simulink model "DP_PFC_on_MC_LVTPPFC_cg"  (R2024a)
settings: Solver=FixedStepDiscrete  StartTime=0.0  StopTime=0.2  FixedStep=10e-6  RelTol=1e-3  EnableMultiTasking=on
model workspace (MAT data in the model file):
  Freq = 100
  Phas = 0
  SinFreq_1 = 250
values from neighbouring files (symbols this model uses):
  ADC = ADCType.Noise    [TotemPole_PFCData.m]
  Control = ControlType.Simple    [TotemPole_PFCData.m]
  Tsc_slow = 0.01    [TotemPole_PFCData.m]
undefined symbols (not defined in the file or in its folder): a, A0, A8, AD1, AD2, AD3, AD4, AD5, address, also, AN11, AN2, AN3, AN5, AN6, AppData, as, B0, B10, B11, B7, B8, below, bin2dec, bit, bits, BOR, C, C6, C7, C9, cause, characters, Code, Communicate, contains, counter, D, D4, Data, data, dead, default, Detailed, deviced, disasserted, DS70005539, dsPIC33AK128MC106, EC, ECIO, ensure, events, Family, faster, Floating, fulll, highest, HS, HS3, I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
libraries: MCHP_Blockset x16, simulink x4, dspswit3 x1
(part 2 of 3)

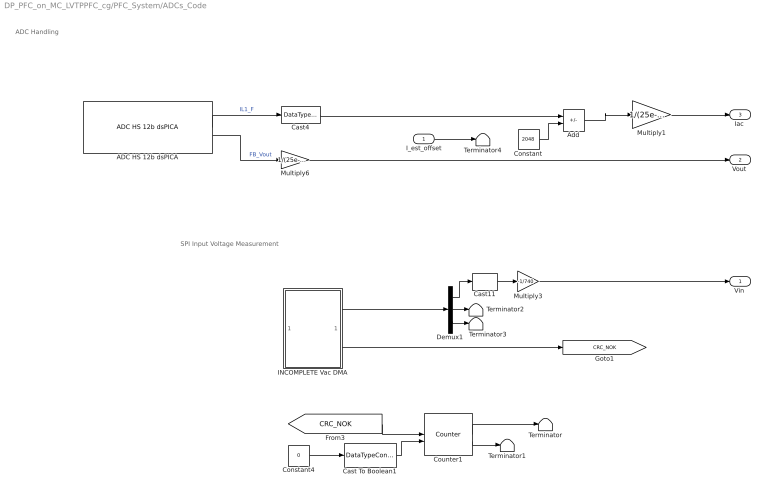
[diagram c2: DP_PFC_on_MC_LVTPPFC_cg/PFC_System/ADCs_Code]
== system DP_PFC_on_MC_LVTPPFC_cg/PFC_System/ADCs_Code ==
  note: ADC Handling
  note: SPI Input Voltage Measurement
  I_est_offset : Inport
  ADC HS 12b dsPICA : MCHP_Blockset/Analog IO/ADC HS 12b dsPICA  ADCREF=ADC 1 and ADC 2  ADC1_refChannel=0 (highest priority)  ADC2_refChannel=0 (highest priority)  ADC3_refChannel=0 (highest priority)  ADC4_refChannel=0 (highest priority)  ADC5_refChannel=Not used  CALRATE=once at startup  VREF_RNG=3.0V to 3.6V  BUFEN=on  info=0  SampleTime=10e-6  MCHP_PORT={ADC1_seq0.0}{ADC1B8}15:2:B8;{ADC2_seq0.0}{ADC2A0}15:2:A0;{ADC1_seq0.0}{ADC1B8}15:2:B8;{ADC2_seq0.0}{ADC2A0}15:2:A0;  MCHP_MASTERLINK=TotemPole_PFC_CodeGen/PFC_System/Control Variant /Microchip Master1  MCHP_CRC=34192788  ADC_Synchronisation=Triggered by custom source  ADC_Trig_TXT=PWM1_Trg1  ADC_TrigTimeStep=on  TrigSource_seq0=Dynamic Options  TrigSource_seq0_TXT=PWM1 adc trig 0  SampleTime_seq0_Tad=Dynamic Options  SampleTime_seq0_Tad_TXT="4.5 Tad  = 56.2ns  -  Rin < 5.2 kOhm"  ADC1_seq0=Dynamic Options  ADC1_seq0_TXT=AD1 AN11 / B8 / Pin[23]  ADC1_seq0_align=Right aligned  ADC1_seq0_overSampling=x1 (12 bits)  ADC2_seq0=Dynamic Options  ADC2_seq0_TXT=AD2 AN6 / A0 / Pin[1]  ADC2_seq0_align=Right aligned  ADC2_seq0_overSampling=x1 (12 bits)  ADC3_seq0=Dynamic Options  ADC3_seq0_TXT=AD3 AN5 / A0 / Pin[1]  ADC3_seq0_align=Left aligned  ADC3_seq0_overSampling=x1 (12 bits)  ADC4_seq0=Dynamic Options  ADC4_seq0_TXT=AD4 AN2 / B7 / Pin[30]  ADC4_seq0_align=Right aligned  ADC4_seq0_overSampling=x256 (16 bits)  ADC5_seq0=Dynamic Options  ADC5_seq0_TXT=AD5 AN3 / A8 / Pin[7]  ADC5_seq0_align=Right aligned  ADC5_seq0_overSampling=x256 (16 bits)  ADC1_seq0_1=Dynamic Options  ADC1_seq0_1_TXT=Not Used  ADC1_seq0_1_align=Right aligned  ADC1_seq0_1_overSampling=x1 (12 bits)  ADC2_seq0_1=Dynamic Options  ADC2_seq0_1_TXT=Not Used  ADC2_seq0_1_align=Right aligned  ADC2_seq0_1_overSampling=x1 (12 bits)  ADC3_seq0_1=Dynamic Options  ADC3_seq0_1_TXT=Not Used  ADC3_seq0_1_align=Right aligned  ADC3_seq0_1_overSampling=x1 (12 bits)  ADC4_seq0_1=Dynamic Options  ADC4_seq0_1_TXT=Not Used  ADC4_seq0_1_align=Right aligned  ADC4_seq0_1_overSampling=x1 (12 bits)  ADC5_seq0_1=Dynamic Options  ADC5_seq0_1_TXT=Not Used  ADC5_seq0_1_align=Right aligned  ADC5_seq0_1_overSampling=x1 (12 bits)  ADC1_seq0_2=Dynamic Options  ADC1_seq0_2_TXT=Not Used  ADC1_seq0_2_align=Right aligned  ADC1_seq0_2_overSampling=x1 (12 bits)  ADC2_seq0_2=Dynamic Options  ADC2_seq0_2_TXT=Not Used  ADC2_seq0_2_align=Right aligned  ADC2_seq0_2_overSampling=x1 (12 bits)  ADC3_seq0_2=Dynamic Options  ADC3_seq0_2_TXT=Not Used  ADC3_seq0_2_align=Right aligned  ADC3_seq0_2_overSampling=x1 (12 bits)  ADC4_seq0_2=Dynamic Options  ADC4_seq0_2_TXT=Not Used  ADC4_seq0_2_align=Right aligned  ADC4_seq0_2_overSampling=x1 (12 bits)  ADC5_seq0_2=Dynamic Options  ADC5_seq0_2_TXT=Not Used  ADC5_seq0_2_align=Right aligned  ADC5_seq0_2_overSampling=x1 (12 bits)  ADC1_seq0_3=Dynamic Options  ADC1_seq0_3_TXT=Not Used  ADC1_seq0_3_align=Right aligned  ADC1_seq0_3_overSampling=x1 (12 bits)  ADC2_seq0_3=Dynamic Options  ADC2_seq0_3_TXT=Not Used  ADC2_seq0_3_align=Right aligned  ADC2_seq0_3_overSampling=x1 (12 bits)  ADC3_seq0_3=Dynamic Options  ADC3_seq0_3_TXT=Not Used  ADC3_seq0_3_align=Right aligned  ADC3_seq0_3_overSampling=x1 (12 bits)  ADC4_seq0_3=Dynamic Options  ADC4_seq0_3_TXT=Not Used  ADC4_seq0_3_align=Right aligned  ADC4_seq0_3_overSampling=x1 (12 bits)  ADC5_seq0_3=Dynamic Options  ADC5_seq0_3_TXT=Not Used  ADC5_seq0_3_align=Right aligned  ADC5_seq0_3_overSampling=x1 (12 bits)  ADC1_seq0_4=Dynamic Options  ADC1_seq0_4_TXT=Not Used  ADC1_seq0_4_align=Right aligned  ADC1_seq0_4_overSampling=x1 (12 bits)  ADC2_seq0_4=Dynamic Options  ADC2_seq0_4_TXT=Not Used  ADC2_seq0_4_align=Right aligned  ADC2_seq0_4_overSampling=x1 (12 bits)  ADC3_seq0_4=Dynamic Options  ADC3_seq0_4_TXT=Not Used  ADC3_seq0_4_align=Right aligned  ADC3_seq0_4_overSampling=x1 (12 bits)  ADC4_seq0_4=Dynamic Options  ADC4_seq0_4_TXT=Not Used  ADC4_seq0_4_align=Right aligned  ADC4_seq0_4_overSampling=x1 (12 bits)  ADC5_seq0_4=Dynamic Options  ADC5_seq0_4_TXT=Not Used  ADC5_seq0_4_align=Right aligned  ADC5_seq0_4_overSampling=x1 (12 bits)  ADC1_seq0_5=Dynamic Options  ADC1_seq0_5_TXT=Not Used  ADC1_seq0_5_align=Right aligned  ADC1_seq0_5_overSampling=x1 (12 bits)  ADC2_seq0_5=Dynamic Options  ADC2_seq0_5_TXT=Not Used  ADC2_seq0_5_align=Right aligned  ADC2_seq0_5_overSampling=x1 (12 bits)  ADC3_seq0_5=Dynamic Options  ADC3_seq0_5_TXT=Not Used  ADC3_seq0_5_align=Right aligned  ADC3_seq0_5_overSampling=x1 (12 bits)  ADC4_seq0_5=Dynamic Options  ADC4_seq0_5_TXT=Not Used  ADC4_seq0_5_align=Right aligned  ADC4_seq0_5_overSampling=x1 (12 bits)  ADC5_seq0_5=Dynamic Options  ADC5_seq0_5_TXT=Not Used  ADC5_seq0_5_align=Right aligned  ADC5_seq0_5_overSampling=x1 (12 bits)  ADC_TRG2_ACCBRST_seq0=Burst - not interruptible  ADC1_NINSEL_seq0=Dynamic Options  ADC1_NINSEL_seq0_TXT=Vss - single ended (unsigned)  ADC2_NINSEL_seq0=Dynamic Options  ADC2_NINSEL_seq0_TXT=Vss - single ended (unsigned)  ADC3_NINSEL_seq0=Dynamic Options  ADC3_NINSEL_seq0_TXT=Vss - single ended (unsigned)  ADC4_NINSEL_seq0=Dynamic Options  ADC4_NINSEL_seq0_TXT=Vss - single ended (unsigned)  ADC5_NINSEL_seq0=Dynamic Options  ADC5_NINSEL_seq0_TXT=Vss - single ended (unsigned)  TrigTimeStep_seq0=on  info_seq0=0  TrigSource_seq1=Dynamic Options  TrigSource_seq1_TXT=after previous sequence  SampleTime_seq1_Tad=Dynamic Options  SampleTime_seq1_Tad_TXT="0.5 Tad  = 6.25ns  -  Rin < 0 kOhm"  ADC1_seq1=Dynamic Options  ADC1_seq1_TXT=Not Used  ADC1_seq1_align=Right aligned  ADC1_seq1_overSampling=x1 (12 bits)  ADC2_seq1=Dynamic Options  ADC2_seq1_TXT=Not Used  ADC2_seq1_align=Right aligned  ADC2_seq1_overSampling=x1 (12 bits)  ADC3_seq1=Dynamic Options  ADC3_seq1_TXT=Not Used  ADC3_seq1_align=Right aligned  ADC3_seq1_overSampling=x1 (12 bits)  ADC4_seq1=Dynamic Options  ADC4_seq1_TXT=Not Used  ADC4_seq1_align=Right aligned  ADC4_seq1_overSampling=x1 (12 bits)  ADC5_seq1=Dynamic Options  ADC5_seq1_TXT=Not Used  ADC5_seq1_align=Right aligned  ADC5_seq1_overSampling=x1 (12 bits)  ADC1_seq1_1=Dynamic Options  ADC1_seq1_1_TXT=Not Used  ADC1_seq1_1_align=Right aligned  ADC1_seq1_1_overSampling=x1 (12 bits)  ADC2_seq1_1=Dynamic Options  ADC2_seq1_1_TXT=Not Used  ADC2_seq1_1_align=Right aligned  ADC2_seq1_1_overSampling=x1 (12 bits)  ADC3_seq1_1=Dynamic Options  ADC3_seq1_1_TXT=Not Used  ADC3_seq1_1_align=Right aligned  ADC3_seq1_1_overSampling=x1 (12 bits)  ADC4_seq1_1=Dynamic Options  ADC4_seq1_1_TXT=Not Used  ADC4_seq1_1_align=Right aligned  ADC4_seq1_1_overSampling=x1 (12 bits)  ADC5_seq1_1=Dynamic Options  ADC5_seq1_1_TXT=Not Used  ADC5_seq1_1_align=Right aligned  ADC5_seq1_1_overSampling=x1 (12 bits)  ADC1_seq1_2=Dynamic Options  ADC1_seq1_2_TXT=Not Used  ADC1_seq1_2_align=Right aligned  ADC1_seq1_2_overSampling=x1 (12 bits)  ADC2_seq1_2=Dynamic Options  ADC2_seq1_2_TXT=Not Used  ADC2_seq1_2_align=Right aligned  ADC2_seq1_2_overSampling=x1 (12 bits)  ADC3_seq1_2=Dynamic Options  ADC3_seq1_2_TXT=Not Used  ADC3_seq1_2_align=Right aligned  ADC3_seq1_2_overSampling=x1 (12 bits)  ADC4_seq1_2=Dynamic Options  ADC4_seq1_2_TXT=Not Used  ADC4_seq1_2_align=Right aligned  ADC4_seq1_2_overSampling=x1 (12 bits)  ADC5_seq1_2=Dynamic Options  ADC5_seq1_2_TXT=Not Used  ADC5_seq1_2_align=Right aligned  ADC5_seq1_2_overSampling=x1 (12 bits)  ADC1_seq1_3=Dynamic Options  ADC1_seq1_3_TXT=Not Used  ADC1_seq1_3_align=Right aligned  ADC1_seq1_3_overSampling=x1 (12 bits)  ADC2_seq1_3=Dynamic Options  ADC2_seq1_3_TXT=Not Used  ADC2_seq1_3_align=Right aligned  ADC2_seq1_3_overSampling=x1 (12 bits)  ADC3_seq1_3=Dynamic Options  ADC3_seq1_3_TXT=Not Used  ADC3_seq1_3_align=Right aligned  ADC3_seq1_3_overSampling=x1 (12 bits)  ADC4_seq1_3=Dynamic Options  ADC4_seq1_3_TXT=Not Used  ADC4_seq1_3_align=Right aligned  ADC4_seq1_3_overSampling=x1 (12 bits)  ADC5_seq1_3=Dynamic Options  ADC5_seq1_3_TXT=Not Used  ADC5_seq1_3_align=Right aligned  ADC5_seq1_3_overSampling=x1 (12 bits)  ADC1_seq1_4=Dynamic Options  ADC1_seq1_4_TXT=Not Used  ADC1_seq1_4_align=Right aligned  ADC1_seq1_4_overSampling=x1 (12 bits)  ADC2_seq1_4=Dynamic Options  ADC2_seq1_4_TXT=Not Used  ADC2_seq1_4_align=Right aligned  ADC2_seq1_4_overSampling=x1 (12 bits)  ADC3_seq1_4=Dynamic Options  ADC3_seq1_4_TXT=Not Used  ADC3_seq1_4_align=Right aligned  ADC3_seq1_4_overSampling=x1 (12 bits)  ADC4_seq1_4=Dynamic Options  ADC4_seq1_4_TXT=Not Used  ADC4_seq1_4_align=Right aligned  ADC4_seq1_4_overSampling=x1 (12 bits)  ADC5_seq1_4=Dynamic Options  ADC5_seq1_4_TXT=Not Used  ADC5_seq1_4_align=Right aligned  ADC5_seq1_4_overSampling=x1 (12 bits)  ADC1_seq1_5=Dynamic Options  ADC1_seq1_5_TXT=Not Used  ADC1_seq1_5_align=Right aligned  ADC1_seq1_5_overSampling=x1 (12 bits)  ADC2_seq1_5=Dynamic Options  ADC2_seq1_5_TXT=Not Used  ADC2_seq1_5_align=Right aligned  ADC2_seq1_5_overSampling=x1 (12 bits)  ADC3_seq1_5=Dynamic Options  ADC3_seq1_5_TXT=Not Used  ADC3_seq1_5_align=Right aligned  ADC3_seq1_5_overSampling=x1 (12 bits)  ADC4_seq1_5=Dynamic Options  ADC4_seq1_5_TXT=Not Used  ADC4_seq1_5_align=Right aligned  ADC4_seq1_5_overSampling=x1 (12 bits)  ADC5_seq1_5=Dynamic Options  ADC5_seq1_5_TXT=Not Used  ADC5_seq1_5_align=Right aligned  ADC5_seq1_5_overSampling=x1 (12 bits)  ADC_TRG2_ACCBRST_seq1=Burst - not interruptible  ADC1_NINSEL_seq1=Dynamic Options  ADC1_NINSEL_seq1_TXT=Vss - single ended (unsigned)  ADC2_NINSEL_seq1=Dynamic Options  ADC2_NINSEL_seq1_TXT=Vss - single ended (unsigned)  ADC3_NINSEL_seq1=Dynamic Options  ADC3_NINSEL_seq1_TXT=Vss - single ended (unsigned)  ADC4_NINSEL_seq1=Dynamic Options  ADC4_NINSEL_seq1_TXT=Vss - single ended (unsigned)  ADC5_NINSEL_seq1=Dynamic Options  ADC5_NINSEL_seq1_TXT=Vss - single ended (unsigned)  TrigTimeStep_seq1=off  info_seq1=0  TrigSource_seq2=Dynamic Options  TrigSource_seq2_TXT=after previous sequence  SampleTime_seq2_Tad=Dynamic Options  SampleTime_seq2_Tad_TXT="0.5 Tad  = 6.25ns  -  Rin < 0 kOhm"  ADC1_seq2=Dynamic Options  ADC1_seq2_TXT=Not Used  ADC1_seq2_align=Right aligned  ADC1_seq2_overSampling=x1 (12 bits)  ADC2_seq2=Dynamic Options  ADC2_seq2_TXT=Not Used  ADC2_seq2_align=Right aligned  ADC2_seq2_overSampling=x1 (12 bits)  ADC3_seq2=Dynamic Options  ADC3_seq2_TXT=Not Used  ADC3_seq2_align=Right aligned  ADC3_seq2_overSampling=x1 (12 bits)  ADC4_seq2=Dynamic Options  ADC4_seq2_TXT=Not Used  ADC4_seq2_align=Right aligned  ADC4_seq2_overSampling=x1 (12 bits)  ADC5_seq2=Dynamic Options  ADC5_seq2_TXT=Not Used  ADC5_seq2_align=Right aligned  ADC5_seq2_overSampling=x1 (12 bits)  ADC1_seq2_1=Dynamic Options  ADC1_seq2_1_TXT=Not Used  ADC1_seq2_1_align=Right aligned  ADC1_seq2_1_overSampling=x1 (12 bits)  ADC2_seq2_1=Dynamic Options  ADC2_seq2_1_TXT=Not Used  ADC2_seq2_1_align=Right aligned  ADC2_seq2_1_overSampling=x1 (12 bits)  ADC3_seq2_1=Dynamic Options  ADC3_seq2_1_TXT=Not Used  ADC3_seq2_1_align=Right aligned  ADC3_seq2_1_overSampling=x1 (12 bits)  ADC4_seq2_1=Dynamic Options  ADC4_seq2_1_TXT=Not Used  ADC4_seq2_1_align=Right aligned  ADC4_seq2_1_overSampling=x1 (12 bits)  ADC5_seq2_1=Dynamic Options  ADC5_seq2_1_TXT=Not Used  ADC5_seq2_1_align=Right aligned  ADC5_seq2_1_overSampling=x1 (12 bits)  ADC1_seq2_2=Dynamic Options  ADC1_seq2_2_TXT=Not Used  ADC1_seq2_2_align=Right aligned  ADC1_seq2_2_overSampling=x1 (12 bits)  ADC2_seq2_2=Dynamic Options  ADC2_seq2_2_TXT=Not Used  ADC2_seq2_2_align=Right aligned  ADC2_seq2_2_overSampling=x1 (12 bits)  ADC3_seq2_2=Dynamic Options  ADC3_seq2_2_TXT=Not Used  ADC3_seq2_2_align=Right aligned  ADC3_seq2_2_overSampling=x1 (12 bits)  ADC4_seq2_2=Dynamic Options  ADC4_seq2_2_TXT=Not Used  ADC4_seq2_2_align=Right aligned  ADC4_seq2_2_overSampling=x1 (12 bits)  ADC5_seq2_2=Dynamic Options  ADC5_seq2_2_TXT=Not Used  ADC5_seq2_2_align=Right aligned  ADC5_seq2_2_overSampling=x1 (12 bits)  ADC1_seq2_3=Dynamic Options  ADC1_seq2_3_TXT=Not Used  ADC1_seq2_3_align=Right aligned  ADC1_seq2_3_overSampling=x1 (12 bits)  ADC2_seq2_3=Dynamic Options  ADC2_seq2_3_TXT=Not Used  ADC2_seq2_3_align=Right aligned  ADC2_seq2_3_overSampling=x1 (12 bits)  ADC3_seq2_3=Dynamic Options  ADC3_seq2_3_TXT=Not Used  ADC3_seq2_3_align=Right aligned  ADC3_seq2_3_overSampling=x1 (12 bits)  ADC4_seq2_3=Dynamic Options  ADC4_seq2_3_TXT=Not Used  ADC4_seq2_3_align=Right aligned  ADC4_seq2_3_overSampling=x1 (12 bits)  ADC5_seq2_3=Dynamic Options  ADC5_seq2_3_TXT=Not Used  ADC5_seq2_3_align=Right aligned  ADC5_seq2_3_overSampling=x1 (12 bits)  ADC1_seq2_4=Dynamic Options  ADC1_seq2_4_TXT=Not Used  ADC1_seq2_4_align=Right aligned  ADC1_seq2_4_overSampling=x1 (12 bits)  ADC2_seq2_4=Dynamic Options  ADC2_seq2_4_TXT=Not Used  ADC2_seq2_4_align=Right aligned  ADC2_seq2_4_overSampling=x1 (12 bits)  ADC3_seq2_4=Dynamic Options  ADC3_seq2_4_TXT=Not Used  ADC3_seq2_4_align=Right aligned  ADC3_seq2_4_overSampling=x1 (12 bits)  ADC4_seq2_4=Dynamic Options  ADC4_seq2_4_TXT=Not Used  ADC4_seq2_4_align=Right aligned  ADC4_seq2_4_overSampling=x1 (12 bits)  ADC5_seq2_4=Dynamic Options  ADC5_seq2_4_TXT=Not Used  ADC5_seq2_4_align=Right aligned  ADC5_seq2_4_overSampling=x1 (12 bits)  ADC1_seq2_5=Dynamic Options  ADC1_seq2_5_TXT=Not Used  ADC1_seq2_5_align=Right aligned  ADC1_seq2_5_overSampling=x1 (12 bits)  ADC2_seq2_5=Dynamic Options  ADC2_seq2_5_TXT=Not Used  ADC2_seq2_5_align=Right aligned  ADC2_seq2_5_overSampling=x1 (12 bits)  ADC3_seq2_5=Dynamic Options  ADC3_seq2_5_TXT=Not Used  ADC3_seq2_5_align=Right aligned  ADC3_seq2_5_overSampling=x1 (12 bits)  ADC4_seq2_5=Dynamic Options  ADC4_seq2_5_TXT=Not Used  ADC4_seq2_5_align=Right aligned  ADC4_seq2_5_overSampling=x1 (12 bits)  ADC5_seq2_5=Dynamic Options  ADC5_seq2_5_TXT=Not Used  ADC5_seq2_5_align=Right aligned  ADC5_seq2_5_overSampling=x1 (12 bits)  ADC_TRG2_ACCBRST_seq2=Burst - not interruptible  ADC1_NINSEL_seq2=Dynamic Options  ADC1_NINSEL_seq2_TXT=Vss - single ended (unsigned)  ADC2_NINSEL_seq2=Dynamic Options  ADC2_NINSEL_seq2_TXT=Vss - single ended (unsigned)  ADC3_NINSEL_seq2=Dynamic Options  ADC3_NINSEL_seq2_TXT=Vss - single ended (unsigned)  ADC4_NINSEL_seq2=Dynamic Options  ADC4_NINSEL_seq2_TXT=Vss - single ended (unsigned)  ADC5_NINSEL_seq2=Dynamic Options  ADC5_NINSEL_seq2_TXT=Vss - single ended (unsigned)  TrigTimeStep_seq2=off  info_seq2=0  TrigSource_seq3=Dynamic Options  TrigSource_seq3_TXT=after previous sequence  SampleTime_seq3_Tad=Dynamic Options  SampleTime_seq3_Tad_TXT="0.5 Tad  = 6.25ns  -  Rin < 0 kOhm"  ADC1_seq3=Dynamic Options  ADC1_seq3_TXT=Not Used  ADC1_seq3_align=Right aligned  ADC1_seq3_overSampling=x1 (12 bits)  ADC2_seq3=Dynamic Options  ADC2_seq3_TXT=Not Used  ADC2_seq3_align=Right aligned  ADC2_seq3_overSampling=x1 (12 bits)  ADC3_seq3=Dynamic Options  ADC3_seq3_TXT=Not Used  ADC3_seq3_align=Right aligned  ADC3_seq3_overSampling=x1 (12 bits)  ADC4_seq3=Dynamic Options  ADC4_seq3_TXT=Not Used  ADC4_seq3_align=Right aligned  ADC4_seq3_overSampling=x1 (12 bits)  ADC5_seq3=Dynamic Options  ADC5_seq3_TXT=Not Used  ADC5_seq3_align=Right aligned  ADC5_seq3_overSampling=x1 (12 bits)  ADC1_seq3_1=Dynamic Options  ADC1_seq3_1_TXT=Not Used  ADC1_seq3_1_align=Right aligned  ADC1_seq3_1_overSampling=x1 (12 bits)  ADC2_seq3_1=Dynamic Options  ADC2_seq3_1_TXT=Not Used  ADC2_seq3_1_align=Right aligned  ADC2_seq3_1_overSampling=x1 (12 bits)  ADC3_seq3_1=Dynamic Options  ADC3_seq3_1_TXT=Not Used  ADC3_seq3_1_align=Right aligned  ADC3_seq3_1_overSampling=x1 (12 bits)  ADC4_seq3_1=Dynamic Options  ADC4_seq3_1_TXT=Not Used  ADC4_seq3_1_align=Right aligned  ADC4_seq3_1_overSampling=x1 (12 bits)  ADC5_seq3_1=Dynamic Options  ADC5_seq3_1_TXT=Not Used  ADC5_seq3_1_align=Right aligned  ADC5_seq3_1_overSampling=x1 (12 bits)  ADC1_seq3_2=Dynamic Options  ADC1_seq3_2_TXT=Not Used  ADC1_seq3_2_align=Right aligned  ADC1_seq3_2_overSampling=x1 (12 bits)  ADC2_seq3_2=Dynamic Options  ADC2_seq3_2_TXT=Not Used  ADC2_seq3_2_align=Right aligned  ADC2_seq3_2_overSampling=x1 (12 bits)  ADC3_seq3_2=Dynamic Options  ADC3_seq3_2_TXT=Not Used  ADC3_seq3_2_align=Right aligned  ADC3_seq3_2_overSampling=x1 (12 bits)  ADC4_seq3_2=Dynamic Options  ADC4_seq3_2_TXT=Not Used  ADC4_seq3_2_align=Right aligned  ADC4_seq3_2_overSampling=x1 (12 bits)  ADC5_seq3_2=Dynamic Options  ADC5_seq3_2_TXT=Not Used  ADC5_seq3_2_align=Right aligned  ADC5_seq3_2_overSampling=x1 (12 bits)  ADC1_seq3_3=Dynamic Options  ADC1_seq3_3_TXT=Not Used  ADC1_seq3_3_align=Right aligned  ADC1_seq3_3_overSampling=x1 (12 bits)  ADC2_seq3_3=Dynamic Options  ADC2_seq3_3_TXT=Not Used  ADC2_seq3_3_align=Right aligned  ADC2_seq3_3_overSampling=x1 (12 bits)  ADC3_seq3_3=Dynamic Options  ADC3_seq3_3_TXT=Not Used  ADC3_seq3_3_align=Right aligned  ADC3_seq3_3_overSampling=x1 (12 bits)  ADC4_seq3_3=Dynamic Options  ADC4_seq3_3_TXT=Not Used  ADC4_seq3_3_align=Right aligned  ADC4_seq3_3_overSampling=x1 (12 bits)  ADC5_seq3_3=Dynamic Options  ADC5_seq3_3_TXT=Not Used  ADC5_seq3_3_align=Right aligned  ADC5_seq3_3_overSampling=x1 (12 bits)  ADC1_seq3_4=Dynamic Options  ADC1_seq3_4_TXT=Not Used  ADC1_seq3_4_align=Right aligned  ADC1_seq3_4_overSampling=x1 (12 bits)  ADC2_seq3_4=Dynamic Options  ADC2_seq3_4_TXT=Not Used  ADC2_seq3_4_align=Right aligned  ADC2_seq3_4_overSampling=x1 (12 bits)  ADC3_seq3_4=Dynamic Options  ADC3_seq3_4_TXT=Not Used  ADC3_seq3_4_align=Right aligned  ADC3_seq3_4_overSampling=x1 (12 bits)  ADC4_seq3_4=Dynamic Options  ADC4_seq3_4_TXT=Not Used  ADC4_seq3_4_align=Right aligned  ADC4_seq3_4_overSampling=x1 (12 bits)  ADC5_seq3_4=Dynamic Options  ADC5_seq3_4_TXT=Not Used  ADC5_seq3_4_align=Right aligned  ADC5_seq3_4_overSampling=x1 (12 bits)  ADC1_seq3_5=Dynamic Options  ADC1_seq3_5_TXT=Not Used  ADC1_seq3_5_align=Right aligned  ADC1_seq3_5_overSampling=x1 (12 bits)  ADC2_seq3_5=Dynamic Options  ADC2_seq3_5_TXT=Not Used  ADC2_seq3_5_align=Right aligned  ADC2_seq3_5_overSampling=x1 (12 bits)  ADC3_seq3_5=Dynamic Options  ADC3_seq3_5_TXT=Not Used  ADC3_seq3_5_align=Right aligned  ADC3_seq3_5_overSampling=x1 (12 bits)  ADC4_seq3_5=Dynamic Options  ADC4_seq3_5_TXT=Not Used  ADC4_seq3_5_align=Right aligned  ADC4_seq3_5_overSampling=x1 (12 bits)  ADC5_seq3_5=Dynamic Options  ADC5_seq3_5_TXT=Not Used  ADC5_seq3_5_align=Right aligned  ADC5_seq3_5_overSampling=x1 (12 bits)  ADC_TRG2_ACCBRST_seq3=Burst - not interruptible  ADC1_NINSEL_seq3=Dynamic Options  ADC1_NINSEL_seq3_TXT=Vss - single ended (unsigned)  ADC2_NINSEL_seq3=Dynamic Options  ADC2_NINSEL_seq3_TXT=Vss - single ended (unsigned)  ADC3_NINSEL_seq3=Dynamic Options  ADC3_NINSEL_seq3_TXT=Vss - single ended (unsigned)  ADC4_NINSEL_seq3=Dynamic Options  ADC4_NINSEL_seq3_TXT=Vss - single ended (unsigned)  ADC5_NINSEL_seq3=Dynamic Options  ADC5_NINSEL_seq3_TXT=Vss - single ended (unsigned)  TrigTimeStep_seq3=off  info_seq3=0  TrigSource_seq4=Dynamic Options  TrigSource_seq4_TXT=after previous sequence  SampleTime_seq4_Tad=Dynamic Options  SampleTime_seq4_Tad_TXT="0.5 Tad  = 6.25ns  -  Rin < 0 kOhm"  ADC1_seq4=Dynamic Options  ADC1_seq4_TXT=Not Used  ADC1_seq4_align=Right aligned  ADC1_seq4_overSampling=x1 (12 bits)  ADC2_seq4=Dynamic Options  ADC2_seq4_TXT=Not Used  ADC2_seq4_align=Right aligned  ADC2_seq4_overSampling=x1 (12 bits)  ADC3_seq4=Dynamic Options  ADC3_seq4_TXT=Not Used  ADC3_seq4_align=Right aligned  ADC3_seq4_overSampling=x1 (12 bits)  ADC4_seq4=Dynamic Options  ADC4_seq4_TXT=Not Used  ADC4_seq4_align=Right aligned  ADC4_seq4_overSampling=x1 (12 bits)  ADC5_seq4=Dynamic Options  ADC5_seq4_TXT=Not Used  ADC5_seq4_align=Right aligned  ADC5_seq4_overSampling=x1 (12 bits)  ADC1_seq4_1=Dynamic Options  ADC1_seq4_1_TXT=Not Used  ADC1_seq4_1_align=Right aligned  ADC1_seq4_1_overSampling=x1 (12 bits)  ADC2_seq4_1=Dynamic Options  ADC2_seq4_1_TXT=Not Used  ADC2_seq4_1_align=Right aligned  ADC2_seq4_1_overSampling=x1 (12 bits)  ADC3_seq4_1=Dynamic Options  ADC3_seq4_1_TXT=Not Used  ADC3_seq4_1_align=Right aligned  ADC3_seq4_1_overSampling=x1 (12 bits)  ADC4_seq4_1=Dynamic Options  ADC4_seq4_1_TXT=Not Used  ADC4_seq4_1_align=Right aligned  ADC4_seq4_1_overSampling=x1 (12 bits)  ADC5_seq4_1=Dynamic Options  ADC5_seq4_1_TXT=Not Used  ADC5_seq4_1_align=Right aligned  ADC5_seq4_1_overSampling=x1 (12 bits)  ADC1_seq4_2=Dynamic Options  ADC1_seq4_2_TXT=Not Used  ADC1_seq4_2_align=Right aligned  ADC1_seq4_2_overSampling=x1 (12 bits)  ADC2_seq4_2=Dynamic Options  ADC2_seq4_2_TXT=Not Used  ADC2_seq4_2_align=Right aligned  ADC2_seq4_2_overSampling=x1 (12 bits)  ADC3_seq4_2=Dynamic Options  ADC3_seq4_2_TXT=Not Used  ADC3_seq4_2_align=Right aligned  ADC3_seq4_2_overSampling=x1 (12 bits)  ADC4_seq4_2=Dynamic Options  ADC4_seq4_2_TXT=Not Used  ADC4_seq4_2_align=Right aligned  ADC4_seq4_2_overSampling=x1 (12 bits)  ADC5_seq4_2=Dynamic Options  ADC5_seq4_2_TXT=Not Used  ADC5_seq4_2_align=Right aligned  ADC5_seq4_2_overSampling=x1 (12 bits)  ADC1_seq4_3=Dynamic Options  ADC1_seq4_3_TXT=Not Used  ADC1_seq4_3_align=Right aligned  ADC1_seq4_3_overSampling=x1 (12 bits)  ADC2_seq4_3=Dynamic Options  ADC2_seq4_3_TXT=Not Used  ADC2_seq4_3_align=Right aligned  ADC2_seq4_3_overSampling=x1 (12 bits)  ADC3_seq4_3=Dynamic Options  ADC3_seq4_3_TXT=Not Used  ADC3_seq4_3_align=Right aligned  ADC3_seq4_3_overSampling=x1 (12 bits)  ADC4_seq4_3=Dynamic Options  ADC4_seq4_3_TXT=Not Used  ADC4_seq4_3_align=Right aligned  ADC4_seq4_3_overSampling=x1 (12 bits)  ADC5_seq4_3=Dynamic Options  ADC5_seq4_3_TXT=Not Used  ADC5_seq4_3_align=Right aligned  ADC5_seq4_3_overSampling=x1 (12 bits)  ADC1_seq4_4=Dynamic Options  ADC1_seq4_4_TXT=Not Used  ADC1_seq4_4_align=Right aligned  ADC1_seq4_4_overSampling=x1 (12 bits)  ADC2_seq4_4=Dynamic Options  ADC2_seq4_4_TXT=Not Used  ADC2_seq4_4_align=Right aligned  ADC2_seq4_4_overSampling=x1 (12 bits)  ADC3_seq4_4=Dynamic Options  ADC3_seq4_4_TXT=Not Used  ADC3_seq4_4_align=Right aligned  ADC3_seq4_4_overSampling=x1 (12 bits)  ADC4_seq4_4=Dynamic Options  ADC4_seq4_4_TXT=Not Used  ADC4_seq4_4_align=Right aligned  ADC4_seq4_4_overSampling=x1 (12 bits)  ADC5_seq4_4=Dynamic Options  ADC5_seq4_4_TXT=Not Used  ADC5_seq4_4_align=Right aligned  ADC5_seq4_4_overSampling=x1 (12 bits)  ADC1_seq4_5=Dynamic Options  ADC1_seq4_5_TXT=Not Used  ADC1_seq4_5_align=Right aligned  ADC1_seq4_5_overSampling=x1 (12 bits)  ADC2_seq4_5=Dynamic Options  ADC2_seq4_5_TXT=Not Used  ADC2_seq4_5_align=Right aligned  ADC2_seq4_5_overSampling=x1 (12 bits)  ADC3_seq4_5=Dynamic Options  ADC3_seq4_5_TXT=Not Used  ADC3_seq4_5_align=Right aligned  ADC3_seq4_5_overSampling=x1 (12 bits)  ADC4_seq4_5=Dynamic Options  ADC4_seq4_5_TXT=Not Used  ADC4_seq4_5_align=Right aligned  ADC4_seq4_5_overSampling=x1 (12 bits)  ADC5_seq4_5=Dynamic Options  ADC5_seq4_5_TXT=Not Used  ADC5_seq4_5_align=Right aligned  ADC5_seq4_5_overSampling=x1 (12 bits)  ADC_TRG2_ACCBRST_seq4=Burst - not interruptible  ADC1_NINSEL_seq4=Dynamic Options  ADC1_NINSEL_seq4_TXT=Vss - single ended (unsigned)  ADC2_NINSEL_seq4=Dynamic Options  ADC2_NINSEL_seq4_TXT=Vss - single ended (unsigned)  ADC3_NINSEL_seq4=Dynamic Options  ADC3_NINSEL_seq4_TXT=Vss - single ended (unsigned)  ADC4_NINSEL_seq4=Dynamic Options  ADC4_NINSEL_seq4_TXT=Vss - single ended (unsigned)  ADC5_NINSEL_seq4=Dynamic Options  ADC5_NINSEL_seq4_TXT=Vss - single ended (unsigned)  TrigTimeStep_seq4=off  info_seq4=0  TrigSource_seq5=Dynamic Options  TrigSource_seq5_TXT=after previous sequence  SampleTime_seq5_Tad=Dynamic Options  SampleTime_seq5_Tad_TXT="0.5 Tad  = 6.25ns  -  Rin < 0 kOhm"  ADC1_seq5=Dynamic Options  ADC1_seq5_TXT=Not Used  ADC1_seq5_align=Right aligned  ADC1_seq5_overSampling=x1 (12 bits)  ADC2_seq5=Dynamic Options  ADC2_seq5_TXT=Not Used  ADC2_seq5_align=Right aligned  ADC2_seq5_overSampling=x1 (12 bits)  ADC3_seq5=Dynamic Options  ADC3_seq5_TXT=Not Used  ADC3_seq5_align=Right aligned  ADC3_seq5_overSampling=x1 (12 bits)  ADC4_seq5=Dynamic Options  ADC4_seq5_TXT=Not Used  ADC4_seq5_align=Right aligned  ADC4_seq5_overSampling=x1 (12 bits)  ADC5_seq5=Dynamic Options  ADC5_seq5_TXT=Not Used  ADC5_seq5_align=Right aligned  ADC5_seq5_overSampling=x1 (12 bits)  ADC1_seq5_1=Dynamic Options  ADC1_seq5_1_TXT=Not Used  ADC1_seq5_1_align=Right aligned  ADC1_seq5_1_overSampling=x1 (12 bits)  ADC2_seq5_1=Dynamic Options  ADC2_seq5_1_TXT=Not Used  ADC2_seq5_1_align=Right aligned  ADC2_seq5_1_overSampling=x1 (12 bits)  ADC3_seq5_1=Dynamic Options  ADC3_seq5_1_TXT=Not Used  ADC3_seq5_1_align=Right aligned  ADC3_seq5_1_overSampling=x1 (12 bits)  ADC4_seq5_1=Dynamic Options  ADC4_seq5_1_TXT=Not Used  ADC4_seq5_1_align=Right aligned  ADC4_seq5_1_overSampling=x1 (12 bits)  ADC5_seq5_1=Dynamic Options  ADC5_seq5_1_TXT=Not Used  ADC5_seq5_1_align=Right aligned  ADC5_seq5_1_overSampling=x1 (12 bits)  ADC1_seq5_2=Dynamic Options  ADC1_seq5_2_TXT=Not Used  ADC1_seq5_2_align=Right aligned  ADC1_seq5_2_overSampling=x1 (12 bits)  ADC2_seq5_2=Dynamic Options  ADC2_seq5_2_TXT=Not Used  ADC2_seq5_2_align=Right aligned  ADC2_seq5_2_overSampling=x1 (12 bits)  ADC3_seq5_2=Dynamic Options  ADC3_seq5_2_TXT=Not Used  ADC3_seq5_2_align=Right aligned  ADC3_seq5_2_overSampling=x1 (12 bits)  ADC4_seq5_2=Dynamic Options  ADC4_seq5_2_TXT=Not Used  ADC4_seq5_2_align=Right aligned  ADC4_seq5_2_overSampling=x1 (12 bits)  ADC5_seq5_2=Dynamic Options  ADC5_seq5_2_TXT=Not Used  ADC5_seq5_2_align=Right aligned  ADC5_seq5_2_overSampling=x1 (12 bits)  ADC1_seq5_3=Dynamic Options  ADC1_seq5_3_TXT=Not Used  ADC1_seq5_3_align=Right aligned  ADC1_seq5_3_overSampling=x1 (12 bits)  ADC2_seq5_3=Dynamic Options  ADC2_seq5_3_TXT=Not Used  ADC2_seq5_3_align=Right aligned  ADC2_seq5_3_overSampling=x1 (12 bits)  ADC3_seq5_3=Dynamic Options  ADC3_seq5_3_TXT=Not Used  ADC3_seq5_3_align=Right aligned  ADC3_seq5_3_overSampling=x1 (12 bits)  ADC4_seq5_3=Dynamic Options  ADC4_seq5_3_TXT=Not Used  ADC4_seq5_3_align=Right aligned  ADC4_seq5_3_overSampling=x1 (12 bits)  ADC5_seq5_3=Dynamic Options  ADC5_seq5_3_TXT=Not Used  ADC5_seq5_3_align=Right aligned  ADC5_seq5_3_overSampling=x1 (12 bits)  ADC1_seq5_4=Dynamic Options  ADC1_seq5_4_TXT=Not Used  ADC1_seq5_4_align=Right aligned  ADC1_seq5_4_overSampling=x1 (12 bits)  ADC2_seq5_4=Dynamic Options  ADC2_seq5_4_TXT=Not Used  ADC2_seq5_4_align=Right aligned  ADC2_seq5_4_overSampling=x1 (12 bits)  ADC3_seq5_4=Dynamic Options  ADC3_seq5_4_TXT=Not Used  ADC3_seq5_4_align=Right aligned  ADC3_seq5_4_overSampling=x1 (12 bits)  ADC4_seq5_4=Dynamic Options  ADC4_seq5_4_TXT=Not Used  ADC4_seq5_4_align=Right aligned  ADC4_seq5_4_overSampling=x1 (12 bits)  ADC5_seq5_4=Dynamic Options  ADC5_seq5_4_TXT=Not Used  ADC5_seq5_4_align=Right aligned  ADC5_seq5_4_overSampling=x1 (12 bits)  ADC1_seq5_5=Dynamic Options  ADC1_seq5_5_TXT=Not Used  ADC1_seq5_5_align=Right aligned  ADC1_seq5_5_overSampling=x1 (12 bits)  ADC2_seq5_5=Dynamic Options  ADC2_seq5_5_TXT=Not Used  ADC2_seq5_5_align=Right aligned  ADC2_seq5_5_overSampling=x1 (12 bits)  ADC3_seq5_5=Dynamic Options  ADC3_seq5_5_TXT=Not Used  ADC3_seq5_5_align=Right aligned  ADC3_seq5_5_overSampling=x1 (12 bits)  ADC4_seq5_5=Dynamic Options  ADC4_seq5_5_TXT=Not Used  ADC4_seq5_5_align=Right aligned  ADC4_seq5_5_overSampling=x1 (12 bits)  ADC5_seq5_5=Dynamic Options  ADC5_seq5_5_TXT=Not Used  ADC5_seq5_5_align=Right aligned  ADC5_seq5_5_overSampling=x1 (12 bits)  ADC_TRG2_ACCBRST_seq5=Burst - not interruptible  ADC1_NINSEL_seq5=Dynamic Options  ADC1_NINSEL_seq5_TXT=Vss - single ended (unsigned)  ADC2_NINSEL_seq5=Dynamic Options  ADC2_NINSEL_seq5_TXT=Vss - single ended (unsigned)  ADC3_NINSEL_seq5=Dynamic Options  ADC3_NINSEL_seq5_TXT=Vss - single ended (unsigned)  ADC4_NINSEL_seq5=Dynamic Options  ADC4_NINSEL_seq5_TXT=Vss - single ended (unsigned)  ADC5_NINSEL_seq5=Dynamic Options  ADC5_NINSEL_seq5_TXT=Vss - single ended (unsigned)  TrigTimeStep_seq5=off  info_seq5=0
  Add : Sum  Inputs=+-
  Cast To Boolean1 : DataTypeConversion  OutDataTypeStr=boolean
  Cast11 : DataTypeConversion  OutDataTypeStr=single
  Cast4 : DataTypeConversion  OutDataTypeStr=single
  Constant : Constant  Value=2048  OutDataTypeStr=single
  Constant4 : Constant  Value=0
  Counter1 : dspswit3/Counter  Direction=Up  CountEvent=Non-zero sample  CounterSize=User defined  MaxCount=8192  InitialCount=0  Output=Count and Hit  HitValue=32  ResetInput=on  SamplesPerFrame=1  Ts=1  CntDtype=uint16  HitDtype=Logical
  Demux1 : Demux  Outputs=3
  INCOMPLETE Vac DMA : Subsystem
  Multiply1 : Gain  Gain=1/(25e-3/3.3*4096)
  Multiply3 : Gain  Gain=-1/740
  Multiply6 : Gain  Gain=1/(25e-3/3.3*4096)  ParamDataTypeStr=single  OutDataTypeStr=single
  Terminator{,1..4} (5 alike) : Terminator
  "Vin " : Outport
  "Vout " : Outport  Port=2
  "Iac " : Outport  Port=3
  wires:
  Multiply3/1 -> "Vin "/1
  Cast4/1 -> Add/1
  Multiply6/1 -> "Vout "/1
  ADC HS 12b dsPICA/1 -> Cast4/1  "IL1_F"
  ADC HS 12b dsPICA/2 -> Multiply6/1  "FB_Vout"
  Counter1/1 -> Terminator/1
  Constant4/1 -> Cast To Boolean1/1
  Cast11/1 -> Multiply3/1
  INCOMPLETE Vac DMA/1(L1 L2 L3) -> Demux1/1
  [CRC_NOK] -> Counter1/1
  Cast To Boolean1/1 -> Counter1/2
  INCOMPLETE Vac DMA/2(SPI_CRC_NOK) -> [CRC_NOK]
  Demux1/1 -> Cast11/1
  Counter1/2 -> Terminator1/1
  Demux1/2 -> Terminator2/1
  Demux1/3 -> Terminator3/1
  Multiply1/1 -> "Iac "/1
  I_est_offset/1 -> Terminator4/1
  Add/1 -> Multiply1/1
  Constant/1 -> Add/2

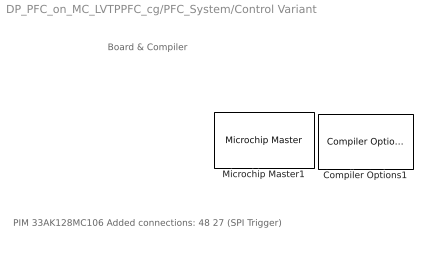
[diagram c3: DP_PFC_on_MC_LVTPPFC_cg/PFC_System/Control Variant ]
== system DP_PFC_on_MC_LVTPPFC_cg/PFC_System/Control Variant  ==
  note: PIM 33AK128MC106 Added connections: 48 27 (SPI Trigger)
  note: Board & Compiler
  Compiler Options1 : MCHP_Blockset/System Configuration/Compiler Options  Priority=1  LATEST_CMPLR=off  COMP_LIST=Dynamic Options  COMP_LIST_TXT=XC-DSC - v3.19  DFP_LIST=Dynamic Options  DFP_LIST_TXT=from compiler  CMSIS_DSP=Dynamic Options  CMSIS_DSP_TXT=Dynamic Options  USE_64BIT_DOUBLE=on  MCHP_MULTITHREAD_COMPILATION=on  UseCustom_LinkerScript=off  MCHP_MASTERLINK=TotemPole_PFC_CodeGen/PFC_System/Control Variant /Microchip Master1  OPTIMIZATION_LEVEL=3  MPLAB_LINKLIB=default  MPLAB_LINKLIB1=default  CodeReplacement=Dynamic Options  CodeReplacement_TXT=None  OPTIMIZATION_FLTO=on  OPTIMIZATION_REORDER=off  OPTIMIZATION_ASM_REORDER=on  UNROLL_LOOPS=off  PROCEDURAL_ABSTRACTION=off  CONSERVE_STACK=off  GC_SECTIONS=None  MCODE=is less than 32768 (faster)  MCONST=in code memory  MDATA=Can use all available memory  MSCALAR=Use only memory below address 8192 (faster)  MLARGEARRAY=off  MAGGREGATE=on  HEAP_SIZE=0  OMF=elf  DEBUG_INFO=on  MCHP_STACK_USAGE=off  GCC_STACK_USAGE=off  ProduceHexOutput=off  AssemblyListing=off  SaveTemps=off  NO_EDS_WARN=on  PRINT_STATISTICS=off
  Microchip Master1 : MCHP_Blockset/System Configuration/Microchip Master  Priority=1  PICREF=33AK128MC106  TIMESTEP_REF=PWM1_Trg1 + ADC  BUSYFLAG=Dynamic Options  BUSYFLAG_TXT=B10 / Pin[31]  VDD_range=Dynamic Options  PWRTEN=Not used  BOREN=Disable  BODENV=2.7V  BORV=Not used  FPWRT=128ms  DSBOREN=Enable ZPBOR during Deep Sleep Mode  DSLPBOR=Not used  MCLRE=Enabled  SMCLR=MCLR pin generates a normal system Reset  PMDL1WAY=Allow only one reconfiguration  RSTPRI=Device will obtain reset instruction from Primary flash  TEMP=Not used  SOSCSRC=Not used  SOSCSEL=Not used  IOL1WAY=Allow only one reconfiguration  ALTVREF=Not used  DISUVREG=Not used  DSSWEN=Not used  LPCFG=Not used  RTCBAT=Not used  VBTBOR=Not used  WUTSEL=Not used  POWERSAVE=off  FNOSC=Primary Oscillator (XT; HS; EC)  FPR=ECIO w/ PLL 16x  FOSFPR=HS3 w/PLL 16x  FOS=Primary Oscillator  FRANGE=High Range  OSCILLATOR_SELECT=External Clock  OSCILLATOR_SELECT_spd=External Clock  QUARTZ=8e6  QUARTZ_spd=8e6  POSCGAIN=2x gain setting  POSCBOOST=Boost the kick start of the oscillator  SOSCGAIN=2x gain setting  SOSCBOOST=Boost the kick start of the oscillator  ACTIV_PLL=on  ACTIV_PLL_spd=on  MIPS_DESIRED=200e6  MIPS_DESIRED_spd=200e6  CPUDIV=Divide by 1  FPLLMUL=Not used  FPLLIDIV=8x Divider  POSCFREQ=Not used  POSCMD=EC (External Clock) Mode  POSCMOD=Primary Oscillator Disabled  MIPS=200 * 1e6  ACLKCON=Optimized for PWM resolution & ADC conversion speed  ACLKCON_spd=Optimized for PWM resolution & ADC conversion speed  FPLLODIV=32x Divider  PLLKEN=PLL lock signal will be used to disable PLL clock output if lock is lost  FCKSM=Both Clock switching and Fail-safe Clock Monitor are enabled  FCKSMEN=Sw Disabled; Mon Disabled  IESO=Start up with FRC; then switch  DSWDTPS=1:2^36  FWDTEN=WDT controlled via SW; use WDTCON.ON bit  FWDTWINSZ=Window size is 25%  FWPSA=1:512  FWPSA0=1:128  FWPSB=1:16  WDT=Disable  WDTPOST=1:32768  WDTPRE=1:128  WDTPS=1:32768  WINDIS=Watchdog Timer operates in Non-Window mode  WWDTEN=Non-Window mode  DSWDTEN=Enable DSWDT during Deep Sleep Mode  DSWDTOSC=Select LPRC as DSWDT Reference clock  FWDT_RCLKSEL=WDT Run Mode uses BFRC:256  FWDT_RWDTPS=1:2147483648  FWDT_SWDTMPS=1:2147483648  FWDT_WDTEN=WDT is controlled by software; use WDTCON.ON bit  FWDT_WDTRSTEN=WDT event generates a reset  FWDT_WDTWIN=WDT Window is 25% of WDT period  FWDT_WINEN=Watchdog Timer operates in Window mode  FPBDIV=Not used  FSOSCEN=Disable Secondary Oscillator  LPRCSEL=Not used  OSCIOFCN=Not used  OSCIOFNC=general purpose digital I/O pin  LVRCFG=Not used  PLL_96MHZ=Not used  PLL96MHZ=Not used  PLLDIV=Not used  WDTCLK=Not used  WDTCMX=Not used  WDTWIN=WDT Window is 25% of WDT period  XTCFG=24-32 MHz crystals  XTBST=Boost the kick-start  APL=Aux Flash Code protect is disabled  APLK=Aux Flash Write Protection or Code Protection is Enabled  AWRP=Auxiliary program memory is not write-protected  BSS=No Protection (other than BWRP)  BWP=Not used  BWRP=Boot Segment may be written  CP=Protection Disabled  EBS=No Boot EEPROM  ESS=No Segment Data EEPROM  GCP=General Segment Code protect is Disabled  GSS=No Protection (other than GWRP)  GSS0=Not used  GSSK=General Segment Write Protection or Code Protection is Enabled  GWRP=General Segment may be written  PWP=Not used  RBS=No Boot RAM  RSS=No Secure RAM  SSS=No Secure Segment  SWRP=Secure segment may be written  WPCFG=Not used  WPDIS=Not used  WPEND=Not used  WPFP=Not used  ICESEL=Communicate on PGEC1/PGED1  ICS=Communicate on PGC2 and PGD2  JTAGEN=Disable  FICD_JTAGEN=Disable  COE=Not used  RES=Not used  DEBUG=Debugger is disabled  BACKBUG=Not used  BKBUG=Not used  ALTI2C=I2C mapped to SDA1/SCL1 pins  ALTI2C1=I2C1 mapped to SDA1/SCL1 pins  ALTI2C2=I2C2 mapped to SDA2/SCL2 pins  ALTI2C3=I2C3 mapped to SDA3/SCL3 pins  FDEVOPT1_ALTI2C1=Not used  FDEVOPT1_ALTI2C2=Not used  FDEVOPT1_SPI2MAPDIS=Not used  FDEVOPT_ALTI2C1=Primary I2C1 pins are used  FDEVOPT_ALTI2C2=Primary I2C2 pins are used  FDEVOPT_ALTI2C3=Primary I2C3 pins are used  FDEVOPT_SPI2PIN=SPI2 pins are selected by peripheral pin selection feature  ALTQIO=QEA1; QEB1; INDX1 are selected as inputs to QEI1  ALTSS1=SS1A is selected as the I/O pin for SPI1  CMPPOL0=Hysteresis is applied to falling edge  CMPPOL1=Hysteresis is applied to falling edge  FCANIO=Not used  FETHIO=Default Ethernet I/O  FMIIEN=MII Enabled  FSRSSEL=Not used  FUSBIDIO=Controlled by the USB Module  FVBUSONIO=Not used  HPOL=PWM module high side output pins have active-high output polarity  HYST0=45 mV Hysteresis  HYST1=45 mV Hysteresis  I2C1SEL=Not used  LPOL=PWM module low side output pins have active-high output polarity  PWMPIN=PWM module pins controlled by PORT register at device Reset  RTCOSC=Not used  UPLLEN=USB PLL Disabled  UPLLIDIV=Not used  ATMOD8=Not used  ALTPMP=Not used  I2C2SEL=Not used  ALTADREF=Not used  ALTCVREF=Not used  PWMLOCK=PWM registers may be written without key sequence  INT_PRIORITY_DMA=0  MCHP_TIMER_RESULT=[ ]  MCHP_PORT={Busy Flag}{Busy}0:1:B10;  MCHP_PLLRegisters="[0        -1     16386        -1  16815713]"  MCHPVAR=MCHP.fcy.MIPS=2e+08;MCHP.fcy.SYSCLK=2e+08;MCHP.fcy.Fplli=8000000;MCHP.fcy.Fvco=1.2e+09;MCHP.fcy.Fpllo=2e+08;MCHP.fcy.PWM=2e+08;MCHP.fcy.ADC=80000000;MCHP.fcy.UART=2e+08;MCHP.fcy.SPI=2e+08;MCHP.fcy.SCC=2e+08;MCHP.fcy.Timers=1e+08;MCHP.fcy.I2C=2e+08;MCHP.PowerSave=0;MCHP.TimeStepFactor=MCHP_Fun.Hex2num('C0F869FFFFFFFFFF');MCHP.TimeStep_Timer=-1;MCHP.NTIMERS=1;MCHP.id.name='33AK128MC106';MCHP.id.N=re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  MCHP_CRC=19172077  BTMODE=Device is in Single Boot (legacy) mode  RES1=Not used  PLLSS=Not used  RES2=Not used  ALTCMPI=Not used  BOREN1=Not used  ALTRB6=Not used  RETCFG=Not used  DFMCY=Not used  BSS2=No Boot Segment  BSEN=No Boot Segment  CWRP=Configuration Segment may be written  CSS=No Protection (other than CWRP)  AIVTDIS=Disabled AIVT  BSLIM=Not used  WDTEN=Disable  BTSWP=BOOTSWP instruction is disabled  DBCC=No Cross Connection between DAC outputs  CTXT1=Not Assigned  CTXT2=Not Assigned  SEQNUM=Not used  nSEQNUM=Not used  BOREN0=Enabled  DMTIVT=Not used  DMTCNT=2^31 (2147483648)  DMTEN=Dead Man Timer is Disabled and can be enabled by software  ON=Not used  USERID=Not used  RESERVED1=Not used  PGL1WAY=Allow only one reconfiguration  FPLLRNG=34-68 MHz Input  FPLLICLK=FRC is input to the System PLL  FPLLMULT=PLL Multiply by 128  UPLLFSEL=USB PLL input is 24 MHz  DMTINTV=Window/Interval value is 127/128 counter value  WDTSPGM=WDT stops during Flash programming  FDMTEN=Deadman Timer is disabled  TRCEN=Trace features in the CPU are enabled  BOOTISA=Boot code and Exception code is MIPS32  FECCCON=ECC and Dynamic ECC are disabled (ECCCON bits are writable)  EXTDDRSIZE=Not used  FSLEEP=Flash is powered down when the device is in Sleep mode  DBGPER=Allow CPU access to all permission regions  EJTAGBEN=Normal EJTAG functionality  TSEQ=Not used  CSEQ=Not used  RWDTPS=1:1048576  RCLKSEL=Always use LPRC  SWDTPS=1:1048576  DMTIVTL=Not used  DMTIVTH=Not used  DMTCNTL=Not used  DMTCNTH=Not used  DMTDIS=Dead Man Timer is Disabled and can be enabled by software  SMBEN=SMBus input threshold is enabled  SPI2PIN=SPI2 uses I/O remap (PPS) pins  CTXT3=Not Assigned  CTXT4=Not Assigned  MBXM0=Mailbox register configured for Main data read (Secondary to Main data transfer)  MBXM1=Mailbox register configured for Main data read (Secondary to Main data transfer)  MBXM2=Mailbox register configured for Main data read (Secondary to Main data transfer)  MBXM3=Mailbox register configured for Main data read (Secondary to Main data transfer)  MBXM4=Mailbox register configured for Main data read (Secondary to Main data transfer)  MBXM5=Mailbox register configured for Main data read (Secondary to Main data transfer)  MBXM6=Mailbox register configured for Main data read (Secondary to Main data transfer)  MBXM7=Mailbox register configured for Main data read (Secondary to Main data transfer)  MBXM8=Mailbox register configured for Main data read (Secondary to Main data transfer)  MBXM9=Mailbox register configured for Main data read (Secondary to Main data transfer)  MBXM10=Mailbox register configured for Main data read (Secondary to Main data transfer)  MBXM11=Mailbox register configured for Main data read (Secondary to Main data transfer)  MBXM12=Mailbox register configured for Main data read (Secondary to Main data transfer)  MBXM13=Mailbox register configured for Main data read (Secondary to Main data transfer)  MBXM14=Mailbox register configured for Main data read (Secondary to Main data transfer)  MBXM15=Mailbox register configured for Main data read (Secondary to Main data transfer)  MBXHSA=MSIxMBXD15 assigned to mailbox handshake protocol block A  MBXHSB=MSIxMBXD15 assigned to mailbox handshake protocol block B  MBXHSC=MSIxMBXD15 assigned to mailbox handshake protocol block C  MBXHSD=MSIxMBXD15 assigned to mailbox handshake protocol block D  MBXHSE=MSIxMBXD15 assigned to mailbox handshake protocol block E  MBXHSF=MSIxMBXD15 assigned to mailbox handshake protocol block F  MBXHSG=MSIxMBXD15 assigned to mailbox handshake protocol block G  MBXHSH=MSIxMBXD15 assigned to mailbox handshake protocol block H  HSAEN=Mailbox data flow control handshake protocol block disabled  HSBEN=Mailbox data flow control handshake protocol block disabled  HSCEN=Mailbox data flow control handshake protocol block disabled  HSDEN=Mailbox data flow control handshake protocol block disabled  HSEEN=Mailbox data flow control handshake protocol block disabled  HSFEN=Mailbox data flow control handshake protocol block disabled  HSGEN=Mailbox data flow control handshake protocol block disabled  HSHEN=Mailbox data flow control handshake protocol block disabled  CPRA0=Main core owns pin  CPRA1=Main core owns pin  CPRA2=Main core owns pin  CPRA3=Main core owns pin  CPRA4=Main core owns pin  CPRB0=Main core owns pin  CPRB1=Main core owns pin  CPRB2=Main core owns pin  CPRB3=Main core owns pin  CPRB4=Main core owns pin  CPRB5=Main core owns pin  CPRB6=Main core owns pin  CPRB7=Main core owns pin  CPRB8=Main core owns pin  CPRB9=Main core owns pin  CPRB10=Main core owns pin  CPRB11=Main core owns pin  CPRB12=Main core owns pin  CPRB13=Main core owns pin  CPRB14=Main core owns pin  CPRB15=Main core owns pin  CPRC0=Main core owns pin  CPRC1=Main core owns pin  CPRC2=Main core owns pin  CPRC3=Main core owns pin  CPRC4=Main core owns pin  CPRC5=Main core owns pin  CPRC6=Main core owns pin  CPRC7=Main core owns pin  CPRC8=Main core owns pin  CPRC9=Main core owns pin  CPRC10=Main core owns pin  CPRC11=Main core owns pin  CPRC12=Main core owns pin  CPRC13=Main core owns pin  CPRC14=Main core owns pin  CPRC15=Main core owns pin  CPRD0=Main core owns pin  CPRD1=Main core owns pin  CPRD2=Main core owns pin  CPRD3=Main core owns pin  CPRD4=Main core owns pin  CPRD5=Main core owns pin  CPRD6=Main core owns pin  CPRD7=Main core owns pin  CPRD8=Main core owns pin  CPRD9=Main core owns pin  CPRD10=Main core owns pin  CPRD11=Main core owns pin  CPRD12=Main core owns pin  CPRD13=Main core owns pin  CPRD14=Main core owns pin  CPRD15=Main core owns pin  CPRE0=Main core owns pin  CPRE1=Main core owns pin  CPRE2=Main core owns pin  CPRE3=Main core owns pin  CPRE4=Main core owns pin  CPRE5=Main core owns pin  CPRE6=Main core owns pin  CPRE7=Main core owns pin  CPRE8=Main core owns pin  CPRE9=Main core owns pin  CPRE10=Main core owns pin  CPRE11=Main core owns pin  CPRE12=Main core owns pin  CPRE13=Main core owns pin  CPRE14=Main core owns pin  CPRE15=Main core owns pin  S1FNOSC=Internal Fast RC (FRC) Oscillator with postscaler  S1IESO=Start up with FRC; then switch  S1OSCIOFNC=OSC2 is clock output  S1FCKSM=Both Clock switching and Fail-safe Clock Monitor are disabled  S1PLLKEN=S1PLLKEN_ON  S1RWDTPS=1:1048576  S1RCLKSEL=Always use LPRC  S1WINDIS=Watchdog Timer operates in Non-Window mode  S1WDTWIN=WDT Window is 25% of WDT period  S1SWDTPS=1:1048576  S1FWDTEN=use WDTCON.ON bit  S1ICS=Communicate on PGC3 and PGD3  S1DEBUG=Not used  S1ISOLAT=The Secondary can operate (in debug mode) even if the SLVEN bit in the MSI is zero  S1NOBTSWP=BOOTSWP instruction is disabled  S1ALTI2C1=I2C1 mapped to SDA1/SCL1 pins  S1SPI1PIN=Secondary SPI1 uses I/O remap (PPS) pins  S1SSRE=Secondary generated resets will reset the Secondary Enable Bit in the MSI module  S1MSRE=The Main software oriented RESET events (RESET Op-Code; Watchdog timeout; TRAP reset; illegalInstruction) will also cause the Secondary subsystem to reset  S1CTXT1=Not Assigned  S1CTXT2=Not Assigned  S1CTXT3=Not Assigned  S1CTXT4=Not Assigned  BORLVL=Not used  BSSO=Not used  MCA=Not used  MAXTEMP=Not used  CFGAN14=Not used  CFGAN15=Not used  S1IOL1WAY=Not used  S1BSSO=Not used  S1BACKBUG=Not used  BISTDIS=mBIST on reset feature disabled  NOBTSWP=BOOTSWP instruction is disabled  S1BISTDIS=Secondary BIST on reset feature disabled  S1DMTIVTL=Not used  S1DMTIVTH=Not used  S1DMTCNTL=Not used  S1DMTCNTH=Not used  S1DMTDIS=Secondary Dead Man Timer is Disabled and can be enabled by software  BSEQ=Not used  IBSEQ=Not used  SMB3EN=SMBus 3.0 input levels  FUSBIDIO2=USBID pin is controlled by the USB2 module  FVBUSIO2=VBUSON pin is controlled by the USB2 module  FUSBIDIO1=USBID pin is controlled by the USB1 module  FVBUSIO1=VBUSON pin is controlled by the USB1 module  VBATBOREN=Enable ZPBOR during VBAT Mode  FDSEN=Enable DSEN bit in DSCON  BORSEL=BOR trip voltage 2.1v (Non-OPAMP deviced operation)  POSCFGAIN=Gain is G3  POSCAGCDLY=Settling time = 25ms x AGCRNG  POSCAGCRNG=Range 1x  POSCAGC=Automatic Gain Control for Oscillator  FDBGWP=Not used
